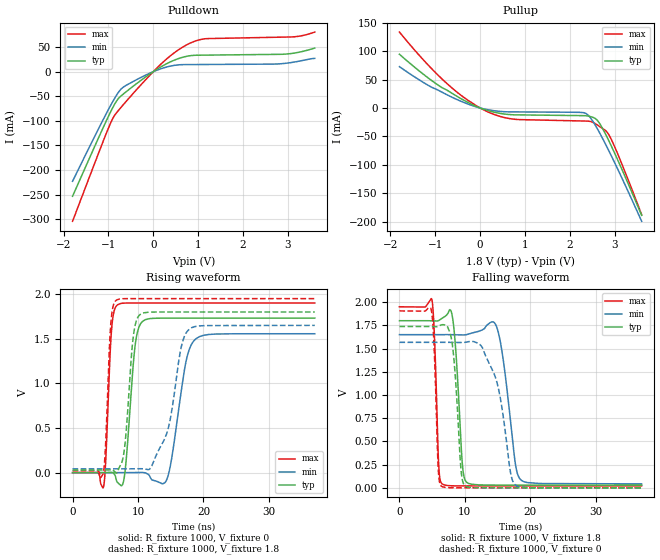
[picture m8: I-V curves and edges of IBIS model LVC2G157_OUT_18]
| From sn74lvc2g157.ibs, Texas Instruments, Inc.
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[Model]   LVC2G157_OUT_18
Model_type  Output
Vref =   0
Rref =   1000
Cref =   30p
Vmeas =   0.9
| variable   typ   min   max
C_comp   9.75pF   6.40pF   16.44pF
| C_pullup   8.77pF   6.40pF   9.59pF
| C_pulldown   10.72pF   6.80pF   16.44pF
[Temperature Range]   40   100   -40
| Ambient temperature   25   85   -40
[Voltage range]   1.8   1.65   1.95
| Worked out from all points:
|   slope of the pulldown table from 0 to 0.27 V, typ, clamps not added: 18.2 ohm
|   slope of the pullup table from 0 to 0.27 V, typ, clamps not added: 41.2 ohm
|   rising waveform, R_fixture 1000, V_fixture 0: 20-80 % time 1.08ns typ, 1.87ns min, 662ps max; typ from 0 V to 1.73 V
|   falling waveform, R_fixture 1000, V_fixture 1.8: 20-80 % time 847ps typ, 1.56ns min, 513ps max; typ from 1.8 V to 0.029 V
|   rising waveform, R_fixture 1000, V_fixture 1.8: 20-80 % time 1.07ns typ, 2.42ns min, 643ps max; typ from 0.029 V to 1.8 V
|   falling waveform, R_fixture 1000, V_fixture 0: 20-80 % time 931ps typ, 2.37ns min, 533ps max; typ from 1.74 V to 0 V
[Pulldown]
| LVC2G157_OUT_18
|   Voltage   I(typ)   I(min)   I(max)
-1.8V     -253.4mA   -222.8mA   -304.2mA
-980mV    -87.07mA   -73.47mA   -110.5mA
-875mV    -68.23mA   -56.15mA   -90.62mA
-735mV    -50.6mA    -37.06mA   -74.26mA
-610mV    -41.17mA   -28.02mA   -60.94mA
-135mV    -8.478mA   -5.492mA   -12.95mA
420mV     21.51mA    12mA       35.04mA
785mV     31.91mA    14.4mA     56.43mA
1.115V    33.57mA    14.58mA    66.41mA
2.935V    35.63mA    16.87mA    70.3mA
3.265V    39.89mA    21.62mA    72.33mA
3.6V      48.06mA    27.06mA    80.56mA
[Pullup]
| LVC2G157_OUT_18
|   Voltage   I(typ)   I(min)   I(max)
-1.8V     94.5mA     72.68mA    133.5mA
-1.175V   53.82mA    40.63mA    76.83mA
-760mV    32.25mA    24.1mA     44.39mA
-340mV    12.65mA    9.054mA    17.33mA
130mV     -3.487mA   -2.355mA   -5.288mA
770mV     -12mA      -6.834mA   -19.8mA
2.37V     -13.77mA   -10.23mA   -22.97mA
2.47V     -15.35mA   -18.5mA    -23.99mA
2.61V     -21.61mA   -36.15mA   -29.68mA
2.87V     -57.86mA   -75.39mA   -47.16mA
3.125V    -101.6mA   -117.2mA   -91.79mA
3.6V      -188.7mA   -199.1mA   -187.5mA
[Ramp]
| LVC2G157_OUT_18
| variable   typ   min   max
dV/dt_r   1.13/1.16E-09   1.01/2.01E-09   1.24/7.15E-10
dV/dt_f   1.13/9.25E-10   1.05/1.74E-09   1.21/5.49E-10
R_load = 1000
[Rising Waveform]
| LVC2G157_OUT_18
R_fixture =   1000
C_fixture =   0
L_fixture =   0
V_fixture =   0
V_fixture_min = 0
V_fixture_max = 0
|   Time   V(typ)   V(min)   V(max)
0s        120.1pV    8.686nV    653.7pV
4.73ns    -24.61uV   2.139uV    -158.9mV
5.945ns   2.058mV    -14.59uV   1.59V
6.89ns    -111.3mV   -7.333uV   1.882V
7.89ns    -57.35mV   -24.13uV   1.899V
9.515ns   1.397V     820.2uV    1.901V
10.72ns   1.696V     1.974mV    1.901V
14.42ns   1.731V     -73.17mV   1.901V
18.87ns   1.731V     1.501V     1.901V
37ns      1.731V     1.556V     1.901V
[Falling Waveform]
| LVC2G157_OUT_18
R_fixture =   1000
C_fixture =   0
L_fixture =   0
V_fixture =   1.8
V_fixture_min = 1.65
V_fixture_max = 1.95
|   Time   V(typ)   V(min)   V(max)
0s        1.8V       1.65V      1.95V
4.97ns    1.799V     1.65V      2.024V
6.005ns   1.802V     1.65V      237.2mV
6.525ns   1.827V     1.65V      41.74mV
8.135ns   1.824V     1.649V     21.81mV
9.61ns    257.9mV    1.647V     20.66mV
10.3ns    57.99mV    1.651V     20.55mV
14.85ns   29.45mV    1.733V     20.47mV
18.59ns   29.18mV    82.88mV    20.47mV
37ns      29.16mV    42.57mV    20.47mV
[Rising Waveform]
| LVC2G157_OUT_18
R_fixture =   1000
C_fixture =   0
L_fixture =   0
V_fixture =   1.8
V_fixture_min = 1.65
V_fixture_max = 1.95
|   Time   V(typ)   V(min)   V(max)
0s        29.14mV    42.51mV    20.46mV
4.665ns   29.13mV    42.51mV    -14.69mV
5.83ns    30.82mV    42.5mV     1.656V
6.69ns    -6.601mV   42.51mV    1.932V
7.845ns   221.9mV    42.51mV    1.949V
9.24ns    1.501V     42.94mV    1.95V
10.31ns   1.771V     43.6mV     1.95V
14.35ns   1.8V       430.9mV    1.95V
17.82ns   1.8V       1.607V     1.95V
37ns      1.8V       1.65V      1.95V
[Falling Waveform]
| LVC2G157_OUT_18
R_fixture =   1000
C_fixture =   0
L_fixture =   0
V_fixture =   0
V_fixture_min = 0
V_fixture_max = 0
|   Time   V(typ)   V(min)   V(max)
0s        1.738V     1.567V     1.905V
4.86ns    1.738V     1.567V     1.919V
5.93ns    1.739V     1.567V     205.4mV
6.42ns    1.756V     1.567V     17.01mV
8.04ns    1.563V     1.566V     806.9uV
9.395ns   203.7mV    1.566V     125uV
10.02ns   22.19mV    1.567V     59.28uV
14.64ns   124.1uV    1.195V     7.304uV
17.73ns   27.56uV    28.09mV    6.836uV
37ns      15.3uV     40.97uV    5.5uV
